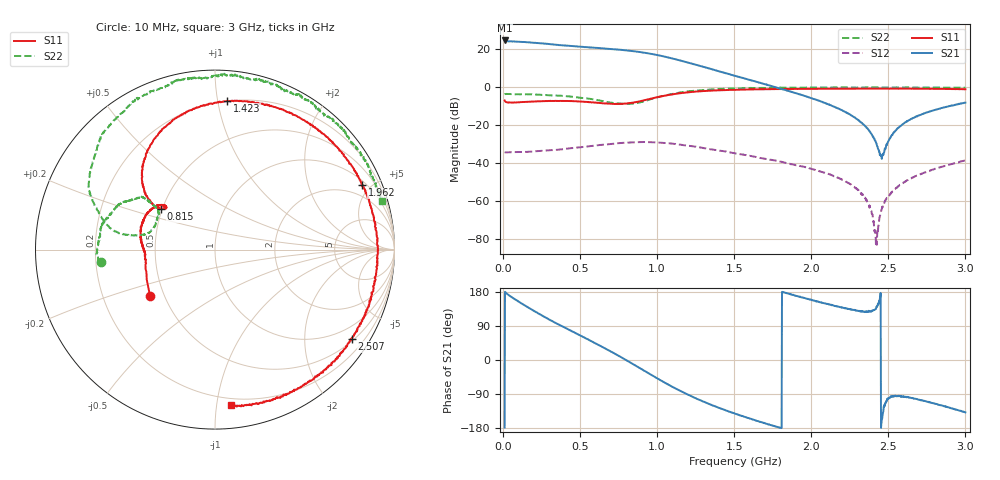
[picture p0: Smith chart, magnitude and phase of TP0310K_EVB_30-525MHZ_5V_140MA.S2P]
!Agilent Technologies,E5071C,MY46523237,B.13.01
!Date: Wed Oct 18 14:11:26 2023
!Data & Calibration Information:
!Freq	S11:SOLT2(ON)	S21:SOLT2(ON)	S12:SOLT2(ON)	S22:SOLT2(ON)
!PortZ  Port1:50+j0  Port2:50+j0
!Above PortZ is port z conversion or system Z0 setting when saving the data.
!When reading, reference impedance value at option line is always used.
# Hz S dB R 50
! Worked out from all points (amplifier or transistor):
!   1197 points, 10 MHz to 3 GHz, reference 50 ohm
!   highest |S21| = 24.6 dB at 10 MHz (marker M1)
!   |S21| within 3 dB of that: start of sweep to 452.4 MHz
!   unconditionally stable (mu >= 1): start of sweep to end of sweep
!   at 507.5 MHz: K = 1.19, MAG = 23.8 dB, |S12| = -31.7 dB
!   at 1.505 GHz: K = 1.40, MAG = 16.7 dB, |S12| = -35.0 dB
!   at 3 GHz: K = 2.37, MAG = 8.7 dB, |S12| = -38.7 dB
!   S11 on the Smith chart (normalised r, x): 10 MHz: 0.42, -0.27; 815 MHz: 0.49, +0.26; 1.423 GHz: 0.20, +1.07; 1.962 GHz: 1.23, +4.45; 2.507 GHz: 0.57, -3.27; 3 GHz: 0.15, -1.10
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1e7  -7.05 -144.6  24.60 -178.3  -34.37 18.2  -3.88 -173.8
5.75e7  -8.21 -175.6  24.17 165.7  -34.40 0.5  -3.72 177.4
1.275e8  -7.94 177.8  23.82 147.2  -34.24 -3.4  -3.80 171.0
2.35e8  -7.51 169.1  23.12 121.4  -33.74 -10.1  -4.05 164.2
3.45e8  -7.27 159.4  22.29 96.6  -33.12 -17.6  -4.46 155.7
5.1e8  -7.63 145.7  21.28 62.7  -31.71 -31.0  -5.71 146.1
5.975e8  -8.21 140.6  20.71 44.4  -30.84 -41.1  -6.58 143.6
6.75e8  -8.67 138.9  20.27 27.8  -30.21 -50.9  -7.86 144.6
8.15e8  -8.50 142.8  19.23 -4.1  -29.27 -72.6  -8.83 158.5
9.2e8  -6.88 142.8  18.09 -29.2  -29.00 -91.7  -7.36 169.4
1.0075e9  -5.21 137.5  16.79 -49.9  -29.26 -108.0  -5.27 170.2
1.0925e9  -3.92 128.3  15.18 -69.6  -29.79 -123.3  -3.73 164.7
1.1975e9  -2.75 114.6  12.96 -91.1  -30.92 -140.5  -2.26 155.1
1.4225e9  -1.60 85.2  7.82 -129.3  -33.70 -171.0  -0.89 133.6
1.505e9  -1.42 75.1  5.97 -141.6  -34.98 179.9  -0.76 126.1
1.9625e9  -0.96 23.6  -4.82 162.7  -42.27 134.7  -0.28 89.7
2.005e9  -0.90 19.2  -5.96 157.6  -43.28 132.6  -0.16 87.0
2.3075e9  -0.83 -12.6  -17.48 129.3  -54.79 106.6  -0.24 64.9
2.42e9  -0.81 -24.2  -29.41 135.1  -83.93 115.6  -0.19 57.5
2.5025e9  -0.82 -32.7  -28.34 -99.9  -57.46 -94.4  -0.27 51.5
2.5075e9  -0.82 -33.1  -27.32 -101.1  -57.15 -97.0  -0.27 51.2
3e9  -1.18 -84.1  -8.23 -138.3  -38.66 -141.9  -0.28 16.3
